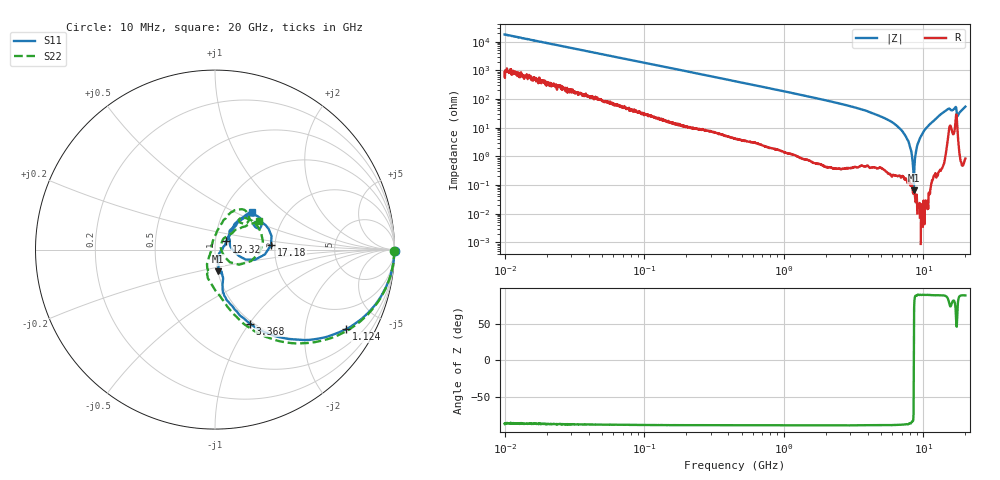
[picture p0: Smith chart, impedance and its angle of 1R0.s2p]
!Keysight Technologies,P5008B,MY61100088,A.16.20.02
!Date: Friday, August 30, 2024 10:49:29
!Correction: S11(C  2-Port  )
!S21(C  2-Port  )
!S12(C  2-Port  )
!S22(C  2-Port  )
!S2P File: Measurements: S11, S21, S12, S22:Log Frequency Sweep
# Hz S  dB  R 50
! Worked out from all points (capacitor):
!   1601 points, 10 MHz to 20 GHz, reference 50 ohm
!   read as one part in series: C = 890 fF near 10.39 MHz
!   lowest |Z| = 65.1 mohm at 8.545 GHz (marker M1)
!   series resonance near 8.548 GHz, so ESL is about 390 pH
!   S11 on the Smith chart (normalised r, x): 10 MHz: open; 1.124 GHz: 1.00, -3.30; 3.368 GHz: 0.97, -1.01; 12.32 GHz: 1.13, +0.10; 17.18 GHz: 1.90, +0.10; 20 GHz: 1.35, +0.63
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1e7  0.00 -0.3  -45.04 86.9  -45.05 87.0  -0.00 -0.3
3.555162e7  -0.01 -1.1  -34.21 87.1  -34.19 87.1  -0.01 -1.2
1.263918e8  -0.03 -4.0  -23.36 85.2  -23.37 85.2  -0.03 -4.1
4.472136e8  -0.26 -13.6  -12.70 75.6  -12.70 75.6  -0.26 -14.1
1.123996e9  -1.36 -31.2  -5.80 57.6  -5.80 57.6  -1.37 -32.7
1.589917e9  -2.43 -41.1  -3.74 47.6  -3.74 47.6  -2.43 -43.1
2.281252e9  -4.13 -52.4  -2.15 36.0  -2.15 36.0  -4.13 -55.1
3.367837e9  -6.81 -64.7  -1.05 23.3  -1.05 23.2  -6.80 -67.8
5.652411e9  -12.22 -79.3  -0.28 6.2  -0.28 6.2  -12.31 -86.7
8.545299e9  -18.20 -81.6  -0.05 -6.8  -0.05 -6.8  -18.33 -108.9
9.854205e9  -21.71 -77.5  0.00 -11.6  0.00 -11.6  -21.82 -120.8
1.099193e10  -28.67 -53.1  0.03 -15.7  0.03 -15.8  -29.99 -145.7
1.13636e10  -29.79 -24.1  0.03 -17.1  0.03 -17.1  -33.01 177.6
1.169216e10  -28.08 0.9  0.02 -18.3  0.02 -18.4  -30.96 135.6
1.231939e10  -22.26 36.2  0.01 -20.6  0.01 -20.7  -23.26 93.3
1.335558e10  -15.61 49.1  -0.07 -25.0  -0.08 -25.1  -15.92 74.7
1.468675e10  -11.41 45.3  -0.40 -31.9  -0.40 -32.0  -11.83 60.2
1.66967e10  -10.90 32.7  -0.89 -36.5  -0.89 -36.6  -12.01 43.2
1.717946e10  -10.10 4.5  -2.37 -33.1  -2.37 -33.2  -12.00 -3.0
1.810106e10  -19.79 42.0  -0.13 -33.9  -0.13 -34.1  -21.15 50.3
1.90721e10  -14.77 52.5  -0.16 -41.4  -0.17 -41.6  -15.06 40.6
2e10  -10.62 46.0  -0.42 -48.3  -0.42 -48.4  -10.75 33.2
